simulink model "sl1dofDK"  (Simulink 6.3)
settings: Solver=ode45  SolverMode=SingleTasking  StartTime=0.0  StopTime=dkt1  RelTol=1e-2  AbsTol=1e-6
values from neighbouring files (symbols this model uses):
  a0 = 1    [runme.m]    (also in gsdata.m = 0)
  a1 = 2    [runme.m]    (also in gsdata.m = 0; getcfactors.m = poly(aRoots1*f)*a(max(size(a))-deg(a)+1))
  a2 = 1    [runme.m]    (also in gsdata.m = 0; getcfactors.m = poly(maxroot(1:maxj)*f))
  a3 = 0    [runme.m]    (also in gsdata.m)
  a_kdk = conv(fdkd,a_kdk)    [Getkdkdp.m]
  b0 = 2    [runme.m]    (also in gsdata.m = 0)
  b1 = 0    [runme.m]    (also in gsdata.m)
  b2 = 0    [runme.m]    (also in gsdata.m)
  b3 = 0    [runme.m]    (also in gsdata.m)
  b_kdk = real(b_kdk)    [Getkdkdp.m]
  dkdst1 = dkdst1tmp    (= 0)    [dkdata.m]    (also in runme.m = 100)
  dkdsv1 = dkdsv1tmp    (= 0)    [dkdata.m]    (also in runme.m = 0.2)
  dkrst1 = dkrst1tmp    (= 0)    [dkdata.m]    (also in runme.m = 1)
  dkrsv1 = dkrsv1tmp    (= 0)    [dkdata.m]    (also in runme.m = 1)
  dkt1 = dkt1tmp    (= 0)    [dkdata.m]    (also in runme.m = 200)
  m0dk = 1    [runme.m]    (also in dkccpe.m = 0)
  m1dk = 0    [runme.m]    (also in dkccpe.m)
  m2dk = 0    [runme.m]    (also in dkccpe.m)
  m3dk = 0    [runme.m]    (also in dkccpe.m)
  r0dk = 1    [runme.m]    (also in dkccpe.m = 0)
  r1dk = 0    [runme.m]    (also in dkccpe.m)
  r2dk = 0    [runme.m]    (also in dkccpe.m)
  r3dk = 0    [runme.m]    (also in dkccpe.m)
  Td = 4    [runme.m]    (also in gsdata.m = 0)

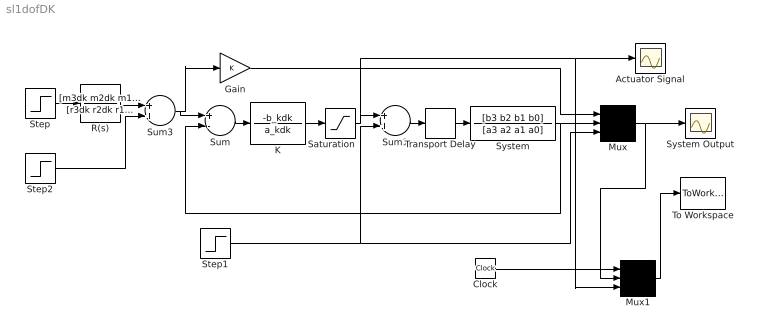
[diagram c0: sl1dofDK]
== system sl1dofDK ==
  Actuator Signal : Scope
  Clock : Clock
  Gain : Gain
  K : TransferFcn  Numerator=-b_kdk  Denominator=a_kdk
  Mux : Mux  Inputs=3
  Mux1 : Mux  Inputs=3
  R(s) : TransferFcn  Numerator=[m3dk m2dk m1dk m0dk]  Denominator=[r3dk r2dk r1dk r0dk]
  Saturation : Saturate  UpperLimit=10  LowerLimit=-10
  Step : Step  Time=dkrst1  After=dkrsv1  SampleTime=0
  Step1 : Step  Time=1200  After=0  SampleTime=0
  Step2 : Step  Time=dkdst1  After=dkdsv1  SampleTime=0
  Sum : Sum  Inputs=+-
  Sum1 : Sum
  Sum3 : Sum
  System : TransferFcn  Numerator=[b3 b2 b1 b0]  Denominator=[a3 a2 a1 a0]
  System Output : Scope
  To Workspace : ToWorkspace  VariableName=o1  SampleTime=dkt1/500  SaveFormat=Array
  Transport Delay : TransportDelay  DelayTime=Td  BufferSize=5000
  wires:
  Sum/1 -> K/1
  Gain/1 -> Mux/1
  Sum1/1 -> Transport Delay/1
  Step1/1 -> Sum1/2, Mux/3
  Mux/1 -> System Output/1, Mux1/2
  Mux1/1 -> To Workspace/1
  Clock/1 -> Mux1/1
  Transport Delay/1 -> System/1
  System/1 -> Mux/2, Sum/2
  Sum3/1 -> Sum/1, Gain/1
  Step2/1 -> Sum3/2
  K/1 -> Saturation/1
  Saturation/1 -> Sum1/1, Actuator Signal/1, Mux1/3
  Step/1 -> R(s)/1
  R(s)/1 -> Sum3/1
